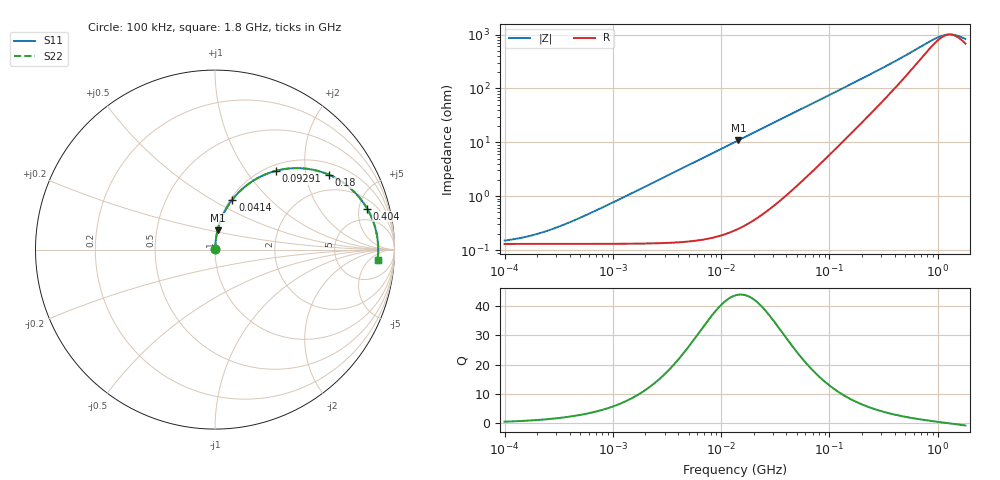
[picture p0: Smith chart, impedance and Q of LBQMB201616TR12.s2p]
! LBQMB201616TR12  S-PARAMETER MODEL  ( General Type )
! Model Generated by TAIYO YUDEN Corporation (http://www.ty-top.com)
! Version 1.0
! TAIYO YUDEN Control No. 191025NI43SB-FBB
! Copyright(c) 2019 TAIYO YUDEN CO.,LTD. All Rights Reserved.
! Product Description (link to TY-COMPAS)
! https://ds.yuden.co.jp/TYCOMPAS/or/detail?pn=LBQMB201616TR12J&u=M
! Products Name : Inductors
! Characteristics :
!  Inductance : 0.12 uH , SRF(min) : 600 MHz , DC Resistance(max) : 0.169 Ohm , Rated Current : 610 mA
!  Case Size : 2.0 x 1.6 / 0.079 x 0.063 [mm/inch] , Thickness : 1.6 / 0.063 [mm/inch]
!  (Conditions: Temperature = 25 degC , DC Bias Current/Voltage = 0A / 0V)
! External Node Assignments :
!  1  o---GGG---o  2
! GND o---------o GND
! Frequency Range : 0.1MHz  -  1800MHz  [ 402 STEP ]
# MHz S RI R 50
! Freq[MHz].  S11 Real  S11 Imag  S21 Real  S21 Imag  S12 Real  S12 Imag  S22 Real  S22 Imag
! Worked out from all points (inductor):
!   401 points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, 100 kHz to 1.8 GHz, reference 50 ohm
!   read as one part in series: L = 120 nH near 528.9 kHz
!   highest Q = 43.9 at 14.44 MHz (marker M1), where L = 120 nH
!   self-resonance near 1.294 GHz
!   S11 on the Smith chart (normalised r, x): 100 kHz: 1.00, +0.00; 41.4 MHz: 1.02, +0.62; 92.91 MHz: 1.10, +1.40; 180 MHz: 1.38, +2.72; 404 MHz: 3.04, +6.06; 1.8 GHz: 15, -9
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0.1  0.0013 0.000752  0.9987 -0.000752  0.9987 -0.000752  0.0013 0.000752
0.144402  0.0013 0.00109  0.9987 -0.00109  0.9987 -0.00109  0.0013 0.00109
0.21369  0.0013 0.00161  0.9987 -0.00161  0.9987 -0.00161  0.0013 0.00161
0.324065  0.0013 0.00244  0.9987 -0.00244  0.9987 -0.00244  0.0013 0.00244
0.516129  0.00131 0.00388  0.9987 -0.00388  0.9987 -0.00388  0.00131 0.00388
2.66389  0.00174 0.02  0.9983 -0.02  0.9983 -0.02  0.00174 0.02
6.593697  0.004 0.0494  0.996 -0.0494  0.996 -0.0494  0.004 0.0494
13.41641  0.0124 0.0997  0.9876 -0.0997  0.9876 -0.0997  0.0124 0.0997
14.43946  0.0141 0.1071  0.9859 -0.1071  0.9859 -0.1071  0.0141 0.1071
25.99364  0.0415 0.1869  0.9585 -0.1869  0.9585 -0.1869  0.0415 0.1869
41.39926  0.097 0.2788  0.903 -0.2788  0.903 -0.2788  0.097 0.2788
69.24595  0.227 0.3924  0.773 -0.3924  0.773 -0.3924  0.227 0.3924
92.90788  0.3412 0.4394  0.6588 -0.4394  0.6588 -0.4394  0.3412 0.4394
127.7465  0.4853 0.453  0.5147 -0.453  0.5147 -0.453  0.4853 0.453
180.0045  0.6351 0.4169  0.3649 -0.4169  0.3649 -0.4169  0.6351 0.4169
253.6402  0.752 0.3436  0.248 -0.3436  0.248 -0.3436  0.752 0.3436
357.3983  0.8288 0.2582  0.1712 -0.2582  0.1712 -0.2582  0.8288 0.2582
403.9647  0.8477 0.2283  0.1523 -0.2283  0.1523 -0.2283  0.8477 0.2283
884.6373  0.9046 0.0656  0.0954 -0.0656  0.0954 -0.0656  0.9046 0.0656
1102.831  0.9085 0.0271  0.0915 -0.0271  0.0915 -0.0271  0.9085 0.0271
1374.841  0.9092 -0.0104  0.0908 0.0104  0.0908 0.0104  0.9092 -0.0104
1800  0.9058 -0.0568  0.0942 0.0568  0.0942 0.0568  0.9058 -0.0568
